| IBIS file stm32u3b5_3c5_wlcsp126.ibs
[IBIS ver] 4.2
[File name] stm32u3b5_3c5_wlcsp126.ibs
[File Rev] 0.1
[Date] 09-03-2026
[Source] Data Created at STMicroelectronics
[Notes]  File originated from ELDO simulations.
[Disclaimer]  This information is for modeling purpose only and is
   not guaranted. The information is subject to change without
   notice.
[Copyright] Copyright 2026 STMicroelectronics Inc.
|   Component stm32u3b5_3c5_wlcsp126
[Component] stm32u3b5_3c5_wlcsp126
[Manufacturer] STMicroelectronics
[Package]
| variable   typ   min   max
R_pkg  0  NA  NA
L_pkg  0  NA  NA
C_pkg  0  NA  NA
[Pin]   signal_name   model_name
A1  VDDUSB  power
A3  VDD  power
A5  PC10  io8_ft_100m_hslv
A7  PD2  io8_ft_100m_hslv
A9  PD6  io8_ft_100m_hslv
A11  VSS  gnd
A13  VDDIO2  power
A15  PB7  io8_ft_100m_hslv
A17  PE0  io8_ft_100m
A19  VDD11  nc
A21  VDD  power
B2  VSS  gnd
B4  PA15  io8_ft_100m
B6  PD1  io8_ft_100m
B8  PD5  io8_ft_100m_hslv
B10  PD7  io8_ft_100m_hslv
B12  PG14  io8_ft_100m_hslv
B14  PB6  io8_ft_100m_hslv
B16  PB9  io8_ft_100m_hslv
B18  PE2  io8_ft_100m
B20  VSS  gnd
C1  PA12  io8usb_ft_phy
C3  PA13  io8_ft_100m
C5  PA14  io8_ft_100m
C7  PD0  io8_ft_100m
C9  PD4  io8_ft_100m_hslv
C11  PG11  io8_ft_100m_hslv
C13  PB4  io8_ft_100m_hslv
C15  PB8  io8_ft_100m_hslv
C17  PC13  io8_ft_100m_v33
C19  PE6  io8_ft_100m
C21  VBAT  power
D2  PA11  io8usb_ft_phy
D4  PA9  io8_ft_100m
D6  PA10  io8_ft_100m
D8  PC12  io8_ft_100m_hslv
D10  PD3  io8_ft_100m_hslv
D12  PG15  io8_ft_100m_hslv
D14  PB5  io8_ft_100m_hslv
D16  PH3-BOOT0  io8_ft_100m_hslv
D18  PE4  io8_ft_100m
D20  PC14-OSC32_IN  io_ft_tamp
E1  PA8  io8_ft_100m_hslv
E3  PC7  io8_ft_100m_hslv
E5  PC8  io8_ft_100m_hslv
E7  PC9  io8_ft_100m_hslv
E9  PC11  io8_ft_100m_hslv
E11  PG12  io8_ft_100m_hslv
E13  PG13  io8_ft_100m_hslv
E15  PB3  io8_ft_100m_hslv
E17  PE3  io8_ft_100m_hslv
E19  PE5  io8_ft_100m
E21  PC15-OSC32_OUT  io_ft_tamp
F2  PC6  io8_ft_100m_hslv
F4  PG6  io8_ft_100m_hslv
F6  PG7  io8_ft_100m_hslv
F8  PG8  io8_ft_100m_hslv
F10  PG9  io8_ft_100m_hslv
F12  PG10  io8_ft_100m_hslv
F14  PF9  io8_ft_100m_hslv
F16  PF8  io8_ft_100m_hslv
F18  PF7  io8_ft_100m_hslv
F20  PF6  io8_ft_100m_hslv
G1  VDDIO2  power
G3  VSS  gnd
G5  PG3  io8_ft_100m_hslv
G7  PG4  io8_ft_100m_hslv
G9  PG5  io8_ft_100m_hslv
G11  PD15  io8_ft_100m
G13  PC1  io8_ft_100m_hslv
G15  PC0  io8_ft_100m_hslv
G17  NRST  ioreset_v33
G19  PF10  io8_ft_100m_hslv
G21  PH0-OSC_IN  io8_ft_100m
H2  PG2  io8_ft_100m_hslv
H4  PD12  io8_ft_100m_hslv
H6  PD14  io8_ft_100m
H8  PB10  io8_ft_100m_hslv
H10  PE15  io8_ft_100m_hslv
H12  PE13  io8_ft_100m_hslv
H14  PE8  io8_ft_100m
H16  PC3  io8_ft_100m_hslv
H18  PC2  io8_ft_100m_hslv
H20  PH1-OSC_OUT  io8_ft_100m
J1  PD13  io8_ft_100m_hslv
J3  PD11  io8_ft_100m_hslv
J5  PD9  io8_ft_100m
J7  PD10  io8_ft_100m
J9  PE14  io8_ft_100m_hslv
J11  PE9  io8_ft_100m_hslv
J13  PB0  io8_ft_100m_hslv
J15  PC4  io8_ft_100m_hslv
J17  PA0  io8_ft_100m
J19  VSSA_VREFM  nc
J21  VREFP  nc
K2  PD8  io8_ft_100m
K4  PB14  io8_ft_100m_hslv
K6  PB12  io8_ft_100m_hslv
K8  PB13  io8_ft_100m_hslv
K10  PE12  io8_ft_100m_hslv
K12  PE7  io8_ft_100m
K14  PC5  io8_ft_100m
K16  PA2  io8_ft_100m_hslv
K18  PA1  io8_ft_100m_hslv
K20  VDDA  nc
L1  PB15  io8_ft_100m
L3  VSS  gnd
L5  VSSSMPS  nc
L7  PB11  io8_ft_100m_hslv
L9  PE11  io8_ft_100m_hslv
L11  VSS  gnd
L13  PB1  io8_ft_100m_hslv
L15  PA6  io8_ft_100m_hslv
L17  PA4  io8_ft_100m_hslv
L19  PA3  io8_ft_100m_hslv
L21  VDD  power
M2  VDD  power
M4  VDD11  nc
M6  VDDSMPS  nc
M8  VLXSMPS  nc
M10  PE10  io8_ft_100m_hslv
M12  VDD  power
M14  PB2  io8_ft_100m_hslv
M16  PA7  io8_ft_100m_hslv
M18  PA5  io8_ft_100m
M20  VSS  gnd
[Package Model]   42a-wlcsp-126-260114
[Pin Mapping]   pulldown_ref   pullup_ref   | Comment
A1  nc  vddusb
A3  nc  vddio
A5  gndio  vddio
A7  gndio  vddio
A9  gndio  vddio
A11  gndio  nc
A13  nc  vddio2
A15  gndio  vddio
A17  gndio  vddio
A19  nc  nc
A21  nc  vddio
B2  gndio  nc
B4  gndio  vddio
B6  gndio  vddio
B8  gndio  vddio
B10  gndio  vddio
B12  gndio  vddio2
B14  gndio  vddio
B16  gndio  vddio
B18  gndio  vddio
B20  gndio  nc
C1  gndio  vddusb  | Depending on IO usage
| C1  gndio  vddio  | Depending on IO usage
C3  gndio  vddio
C5  gndio  vddio
C7  gndio  vddio
C9  gndio  vddio
C11  gndio  vddio2
C13  gndio  vddio
C15  gndio  vddio
C17  gndio  vsw
C19  gndio  vddio
C21  nc  vsw
D2  gndio  vddusb  | Depending on IO usage
| D2  gndio  vddio  | Depending on IO usage
D4  gndio  vddio
D6  gndio  vddio
D8  gndio  vddio
D10  gndio  vddio
D12  gndio  vddio2
D14  gndio  vddio
D16  gndio  vddio
D18  gndio  vddio
D20  gndio  vsw
E1  gndio  vddio
E3  gndio  vddio
E5  gndio  vddio
E7  gndio  vddio
E9  gndio  vddio
E11  gndio  vddio2
E13  gndio  vddio2
E15  gndio  vddio
E17  gndio  vddio
E19  gndio  vddio
E21  gndio  vsw
F2  gndio  vddio
F4  gndio  vddio2
F6  gndio  vddio2
F8  gndio  vddio2
F10  gndio  vddio2
F12  gndio  vddio2
F14  gndio  vddio
F16  gndio  vddio
F18  gndio  vddio
F20  gndio  vddio
G1  nc  vddio2
G3  gndio  nc
G5  gndio  vddio2
G7  gndio  vddio2
G9  gndio  vddio2
G11  gndio  vddio
G13  gndio  vddio
G15  gndio  vddio
G17  gndio  vddio
G19  gndio  vddio
G21  gndio  vddio
H2  gndio  vddio2
H4  gndio  vddio
H6  gndio  vddio
H8  gndio  vddio
H10  gndio  vddio
H12  gndio  vddio
H14  gndio  vddio
H16  gndio  vddio
H18  gndio  vddio
H20  gndio  vddio
J1  gndio  vddio
J3  gndio  vddio
J5  gndio  vddio
J7  gndio  vddio
J9  gndio  vddio
J11  gndio  vddio
J13  gndio  vddio
J15  gndio  vddio
J17  gndio  vddio
J19  nc  nc
J21  nc  nc
K2  gndio  vddio
K4  gndio  vddio
K6  gndio  vddio
K8  gndio  vddio
K10  gndio  vddio
K12  gndio  vddio
K14  gndio  vddio
K16  gndio  vddio
K18  gndio  vddio
K20  nc  nc
L1  gndio  vddio
L3  gndio  nc
L5  nc  nc
L7  gndio  vddio
L9  gndio  vddio
L11  gndio  nc
L13  gndio  vddio
L15  gndio  vddio
L17  gndio  vddio
L19  gndio  vddio
L21  nc  vddio
M2  nc  vddio
M4  nc  nc
M6  nc  nc
M8  nc  nc
M10  gndio  vddio
M12  nc  vddio
M14  gndio  vddio
M16  gndio  vddio
M18  gndio  vddio
M20  gndio  nc
|[Diff Pin]  inv_pin  vdiff  tdelay_typ  tdelay_min  tdelay_max
|C1  D2  NA  NA  NA  NA
[Model Selector] io8_ft_100m
io8_ft_100m_ls_1v2  "GPIO 100MHz - 5V tolerant - low speed - 1.2V range"
io8_ft_100m_ls_1v8  "GPIO 100MHz - 5V tolerant - low speed - 1.8V range"
io8_ft_100m_ls_3v3  "GPIO 100MHz - 5V tolerant - low speed - 3.3V range"
io8_ft_100m_ms_1v2  "GPIO 100MHz - 5V tolerant - med speed - 1.2V range"
io8_ft_100m_ms_1v8  "GPIO 100MHz - 5V tolerant - med speed - 1.8V range"
io8_ft_100m_ms_3v3  "GPIO 100MHz - 5V tolerant - med speed - 3.3V range"
io8_ft_100m_fs_1v2  "GPIO 100MHz - 5V tolerant - fast speed - 1.2V range"
io8_ft_100m_fs_1v8  "GPIO 100MHz - 5V tolerant - fast speed - 1.8V range"
io8_ft_100m_fs_3v3  "GPIO 100MHz - 5V tolerant - fast speed - 3.3V range"
io8_ft_100m_hs_1v2  "GPIO 100MHz - 5V tolerant - high speed - 1.2V range"
io8_ft_100m_hs_1v8  "GPIO 100MHz - 5V tolerant - high speed - 1.8V range"
io8_ft_100m_hs_3v3  "GPIO 100MHz - 5V tolerant - high speed - 3.3V range"
[Model Selector] io8_ft_100m_hslv
io8_ft_100m_ls_1v2  "GPIO 100MHz - 5V tolerant - low speed - 1.2V range"
io8_ft_100m_ls_1v8  "GPIO 100MHz - 5V tolerant - low speed - 1.8V range"
io8_ft_100m_ls_3v3  "GPIO 100MHz - 5V tolerant - low speed - 3.3V range"
io8_ft_100m_ms_1v2  "GPIO 100MHz - 5V tolerant - med speed - 1.2V range"
io8_ft_100m_ms_1v8  "GPIO 100MHz - 5V tolerant - med speed - 1.8V range"
io8_ft_100m_ms_3v3  "GPIO 100MHz - 5V tolerant - med speed - 3.3V range"
io8_ft_100m_fs_1v2  "GPIO 100MHz - 5V tolerant - fast speed - 1.2V range"
io8_ft_100m_fs_1v8  "GPIO 100MHz - 5V tolerant - fast speed - 1.8V range"
io8_ft_100m_fs_3v3  "GPIO 100MHz - 5V tolerant - fast speed - 3.3V range"
io8_ft_100m_hs_1v2  "GPIO 100MHz - 5V tolerant - high speed - 1.2V range"
io8_ft_100m_hs_1v8  "GPIO 100MHz - 5V tolerant - high speed - 1.8V range"
io8_ft_100m_hs_3v3  "GPIO 100MHz - 5V tolerant - high speed - 3.3V range"
io8_ft_100m_hslv_ls_1v2  "GPIO 100MHz low voltage optimization - 5V tolerant - low speed - 1.2V range"
io8_ft_100m_hslv_ls_1v8  "GPIO 100MHz low voltage optimization - 5V tolerant - low speed - 1.8V range"
io8_ft_100m_hslv_ls_2v5  "GPIO 100MHz low voltage optimization - 5V tolerant - low speed - 3.3V range"
io8_ft_100m_hslv_ms_1v2  "GPIO 100MHz low voltage optimization - 5V tolerant - med speed - 1.2V range"
io8_ft_100m_hslv_ms_1v8  "GPIO 100MHz low voltage optimization - 5V tolerant - med speed - 1.8V range"
io8_ft_100m_hslv_ms_2v5  "GPIO 100MHz low voltage optimization - 5V tolerant - med speed - 3.3V range"
io8_ft_100m_hslv_fs_1v2  "GPIO 100MHz low voltage optimization - 5V tolerant - fast speed - 1.2V range"
io8_ft_100m_hslv_fs_1v8  "GPIO 100MHz low voltage optimization - 5V tolerant - fast speed - 1.8V range"
io8_ft_100m_hslv_fs_2v5  "GPIO 100MHz low voltage optimization - 5V tolerant - fast speed - 3.3V range"
io8_ft_100m_hslv_hs_1v2  "GPIO 100MHz low voltage optimization - 5V tolerant - high speed - 1.2V range"
io8_ft_100m_hslv_hs_1v8  "GPIO 100MHz low voltage optimization - 5V tolerant - high speed - 1.8V range"
io8_ft_100m_hslv_hs_2v5  "GPIO 100MHz low voltage optimization - 5V tolerant - high speed - 3.3V range"
[Model Selector] io8_ft_100m_v33
io8_ft_100m_v33_ls_1v2  "GPIO_V33 100MHz - 5V tolerant - low speed - 1.2V range"
io8_ft_100m_v33_ls_1v8  "GPIO_V33 100MHz - 5V tolerant - low speed - 1.8V range"
io8_ft_100m_v33_ls_3v3  "GPIO_V33 100MHz - 5V tolerant - low speed - 3.3V range"
io8_ft_100m_v33_ms_1v2  "GPIO_V33 100MHz - 5V tolerant - med speed - 1.2V range"
io8_ft_100m_v33_ms_1v8  "GPIO_V33 100MHz - 5V tolerant - med speed - 1.8V range"
io8_ft_100m_v33_ms_3v3  "GPIO_V33 100MHz - 5V tolerant - med speed - 3.3V range"
io8_ft_100m_v33_fs_1v2  "GPIO_V33 100MHz - 5V tolerant - fast speed - 1.2V range"
io8_ft_100m_v33_fs_1v8  "GPIO_V33 100MHz - 5V tolerant - fast speed - 1.8V range"
io8_ft_100m_v33_fs_3v3  "GPIO_V33 100MHz - 5V tolerant - fast speed - 3.3V range"
io8_ft_100m_v33_hs_1v2  "GPIO_V33 100MHz - 5V tolerant - high speed - 1.2V range"
io8_ft_100m_v33_hs_1v8  "GPIO_V33 100MHz - 5V tolerant - high speed - 1.8V range"
io8_ft_100m_v33_hs_3v3  "GPIO_V33 100MHz - 5V tolerant - high speed - 3.3V range"
[Model Selector] io8usb_ft_phy
io8_ft_100m_ls_1v2  "GPIO 100MHz - 5V tolerant - low speed - 1.2V range"
io8_ft_100m_ls_1v8  "GPIO 100MHz - 5V tolerant - low speed - 1.8V range"
io8_ft_100m_ls_3v3  "GPIO 100MHz - 5V tolerant - low speed - 3.3V range"
io8_ft_100m_ms_1v2  "GPIO 100MHz - 5V tolerant - med speed - 1.2V range"
io8_ft_100m_ms_1v8  "GPIO 100MHz - 5V tolerant - med speed - 1.8V range"
io8_ft_100m_ms_3v3  "GPIO 100MHz - 5V tolerant - med speed - 3.3V range"
io8_ft_100m_fs_1v2  "GPIO 100MHz - 5V tolerant - fast speed - 1.2V range"
io8_ft_100m_fs_1v8  "GPIO 100MHz - 5V tolerant - fast speed - 1.8V range"
io8_ft_100m_fs_3v3  "GPIO 100MHz - 5V tolerant - fast speed - 3.3V range"
io8_ft_100m_hs_1v2  "GPIO 100MHz - 5V tolerant - high speed - 1.2V range"
io8_ft_100m_hs_1v8  "GPIO 100MHz - 5V tolerant - high speed - 1.8V range"
io8_ft_100m_hs_3v3  "GPIO 100MHz - 5V tolerant - high speed - 3.3V range"
io8usb_ft_phy_hs_3v3   "USB full speed"
io8usb_ft_phy_ls_3v3   "USB low speed"
[Model Selector] io_ft_tamp
io_ft_tamp_ls_1v2 "io8_ft tamp low speed @ 1.2V"
io_ft_tamp_ls_1v8 "io8_ft tamp low speed @ 1.8V"
io_ft_tamp_ls_3v3 "io8_ft tamp low speed @ 3.3V"
io_ft_tamp_ms_1v2 "io8_ft tamp med speed @ 1.2V"
io_ft_tamp_ms_1v8 "io8_ft tamp med speed @ 1.8V"
io_ft_tamp_ms_3v3 "io8_ft tamp med speed @ 3.3V"
io_ft_tamp_fs_1v2 "io8_ft tamp fast speed @ 1.2V"
io_ft_tamp_fs_1v8 "io8_ft tamp fast speed @ 1.8V"
io_ft_tamp_fs_3v3 "io8_ft tamp fast speed @ 3.3V"
io_ft_tamp_hs_1v2 "io8_ft tamp high speed @ 1.2V"
io_ft_tamp_hs_1v8 "io8_ft tamp high speed @ 1.8V"
io_ft_tamp_hs_3v3 "io8_ft tamp high speed @ 3.3V"
[Model Selector] ioreset_v33
ioreset_v33_1v2 "Reset PAD. 5V tolerant. 1.2V range"
ioreset_v33_1v8 "Reset PAD. 5V tolerant. 1.8V range"
ioreset_v33_3v3 "Reset PAD. 5V tolerant. 3.3V range"
[Define Package Model]  42a-wlcsp-126-260114
[Manufacturer]  Unknown
[OEM]  Unknown
[Description]  None
[Number Of Pins]  119
[Pin Numbers]
| Pin Num   Terminal Name
G17 | NRST
J17 | PA0
K18 | PA1
K16 | PA2
L19 | PA3
L17 | PA4
M18 | PA5
L15 | PA6
M16 | PA7
E1 | PA8
D4 | PA9
D6 | PA10
D2 | PA11
C1 | PA12
C3 | PA13
C5 | PA14
B4 | PA15
J13 | PB0
L13 | PB1
M14 | PB2
E15 | PB3
C13 | PB4
D14 | PB5
B14 | PB6
A15 | PB7
C15 | PB8
B16 | PB9
H8 | PB10
L7 | PB11
K6 | PB12
K8 | PB13
K4 | PB14
L1 | PB15
G15 | PC0
G13 | PC1
H18 | PC2
H16 | PC3
J15 | PC4
K14 | PC5
F2 | PC6
E3 | PC7
E5 | PC8
E7 | PC9
A5 | PC10
E9 | PC11
D8 | PC12
C17 | PC13
D20 | PC14-OSC32_IN
E21 | PC15-OSC32_OUT
C7 | PD0
B6 | PD1
A7 | PD2
D10 | PD3
C9 | PD4
B8 | PD5
A9 | PD6
B10 | PD7
K2 | PD8
J5 | PD9
J7 | PD10
J3 | PD11
H4 | PD12
J1 | PD13
H6 | PD14
G11 | PD15
A17 | PE0
B18 | PE2
E17 | PE3
D18 | PE4
E19 | PE5
C19 | PE6
K12 | PE7
H14 | PE8
J11 | PE9
M10 | PE10
L9 | PE11
K10 | PE12
H12 | PE13
J9 | PE14
H10 | PE15
F20 | PF6
F18 | PF7
F16 | PF8
F14 | PF9
G19 | PF10
H2 | PG2
G5 | PG3
G7 | PG4
G9 | PG5
F4 | PG6
F6 | PG7
F8 | PG8
F10 | PG9
F12 | PG10
C11 | PG11
E11 | PG12
E13 | PG13
B12 | PG14
D12 | PG15
G21 | PH0-OSC_IN
H20 | PH1-OSC_OUT
D16 | PH3-BOOT0
M4 | VDD11
A19 | VDD11
C21 | VBAT
A3 | VDD
A21 | VDD
L21 | VDD
M2 | VDD
K20 | VDDA
G1 | VDDIO2
A13 | VDDIO2
M6 | VDDSMPS
A1 | VDDUSB
M8 | VLXSMPS
J21 | VREFP
A11 | VSS
J19 | VSSA_VREFM
L5 | VSSSMPS
|[Merged Pins]  L21
|M12  |  VDD
|[Merged Pins]  A11
|B2  |  VSS
|B20  |  VSS
|G3  |  VSS
|L3  |  VSS
|L11  |  VSS
|M20  |  VSS
[Model Data]
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[End Model Data]
[End Package Model]
|End [Component]
| Models and submodels in the file (53): io8_ft_100m_fs_1v2 (I/O), io8_ft_100m_fs_1v8 (I/O), io8_ft_100m_fs_3v3 (I/O), io8_ft_100m_hs_1v2 (I/O), io8_ft_100m_hs_1v8 (I/O), io8_ft_100m_hs_3v3 (I/O), io8_ft_100m_hslv_fs_1v2 (I/O), io8_ft_100m_hslv_fs_1v8 (I/O), io8_ft_100m_hslv_fs_2v5 (I/O), io8_ft_100m_hslv_hs_1v2 (I/O), io8_ft_100m_hslv_hs_1v8 (I/O), io8_ft_100m_hslv_hs_2v5 (I/O), io8_ft_100m_hslv_ls_1v2 (I/O), io8_ft_100m_hslv_ls_1v8 (I/O), io8_ft_100m_hslv_ls_2v5 (I/O), io8_ft_100m_hslv_ms_1v2 (I/O), io8_ft_100m_hslv_ms_1v8 (I/O), io8_ft_100m_hslv_ms_2v5 (I/O), io8_ft_100m_ls_1v2 (I/O), io8_ft_100m_ls_1v8 (I/O), io8_ft_100m_ls_3v3 (I/O), io8_ft_100m_ms_1v2 (I/O), io8_ft_100m_ms_1v8 (I/O), io8_ft_100m_ms_3v3 (I/O), io8_ft_100m_v33_fs_1v2 (I/O), io8_ft_100m_v33_fs_1v8 (I/O), io8_ft_100m_v33_fs_3v3 (I/O), io8_ft_100m_v33_hs_1v2 (I/O), io8_ft_100m_v33_hs_1v8 (I/O), io8_ft_100m_v33_hs_3v3 (I/O), io8_ft_100m_v33_ls_1v2 (I/O), io8_ft_100m_v33_ls_1v8 (I/O), io8_ft_100m_v33_ls_3v3 (I/O), io8_ft_100m_v33_ms_1v2 (I/O), io8_ft_100m_v33_ms_1v8 (I/O), io8_ft_100m_v33_ms_3v3 (I/O), io8usb_ft_phy_hs_3v3 (I/O), io8usb_ft_phy_ls_3v3 (I/O), io_ft_tamp_fs_1v2 (I/O), io_ft_tamp_fs_1v8 (I/O), io_ft_tamp_fs_3v3 (I/O), io_ft_tamp_hs_1v2 (I/O), io_ft_tamp_hs_1v8 (I/O), io_ft_tamp_hs_3v3 (I/O), io_ft_tamp_ls_1v2 (I/O), io_ft_tamp_ls_1v8 (I/O), io_ft_tamp_ls_3v3 (I/O), io_ft_tamp_ms_1v2 (I/O), io_ft_tamp_ms_1v8 (I/O), io_ft_tamp_ms_3v3 (I/O), ioreset_v33_1v2 (I/O_open_drain), ioreset_v33_1v8 (I/O_open_drain), ioreset_v33_3v3 (I/O_open_drain)
